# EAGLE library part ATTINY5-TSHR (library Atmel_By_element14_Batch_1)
Microcontroller
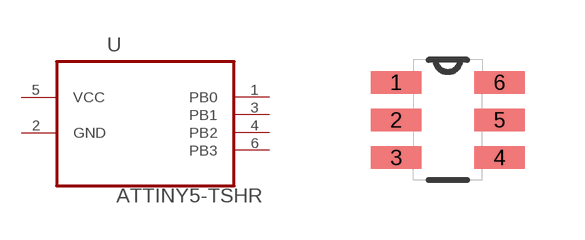
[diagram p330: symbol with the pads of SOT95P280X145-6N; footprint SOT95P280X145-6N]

Designator prefix U

## ATTINY5-TSHR (DESCRIPTION: Microcontroller; MPN: ATTINY5-TSHR; OC_FARNELL: 1841626; OC_NEWARK: 12T1342; PACKAGE: SOT563-6; SUPPLIER: ATMEL)  [SOT95P280X145-6N]
1  PB0
2  GND  pas
3  PB1
4  PB2
5  VCC  pwr
6  PB3

## Footprint SOT95P280X145-6N (pad centres in mm)
smd 1.27 x 0.559: 1 -1.295,0.94; 2 -1.295,0; 3 -1.295,-0.94; 4 1.295,-0.94; 5 1.295,0; 6 1.295,0.94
